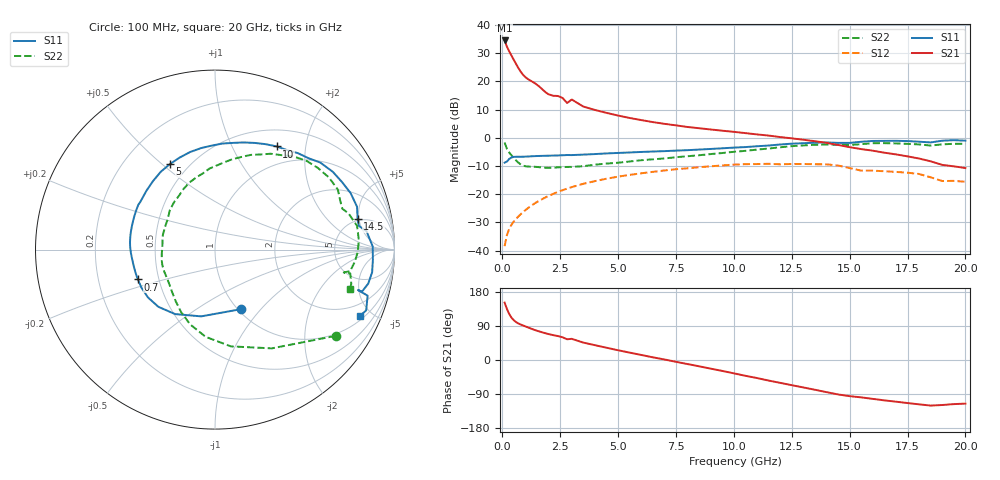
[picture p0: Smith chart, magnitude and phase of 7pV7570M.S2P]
! Infineon Technologies  Discrete & RF Semiconductors
! bfp620
! VCE = 0.75 V,  IC =  70 mA
! Common Emitter S-Parameters:  Sep 2002
# GHz  S  MA  R  50
!  f  S11  S21  S12  S22
! GHz  MAG  ANG  MAG  ANG  MAG  ANG  MAG  ANG
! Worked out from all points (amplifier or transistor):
!   59 points, 100 MHz to 20 GHz, reference 50 ohm
!   highest |S21| = 34.5 dB at 100 MHz (marker M1)
!   |S21| within 3 dB of that: start of sweep to 246.9 MHz
!   unconditionally stable (mu >= 1): 1.803 GHz to 2.397 GHz; 3.082 GHz to 10.85 GHz; 16.75 GHz to end of sweep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
!   at 1 GHz: K = 0.92, MSG = 23.6 dB, |S12| = -25.6 dB
!   at 5.5 GHz: K = 1.06, MAG = 8.6 dB, |S12| = -13.1 dB
!   at 20 GHz: K = 1.55, MAG = -1.9 dB, |S12| = -15.6 dB
!   S11 on the Smith chart (normalised r, x): 100 MHz: 1.03, -0.79; 700 MHz: 0.38, -0.16; 5 GHz: 0.40, +0.53; 10 GHz: 0.72, +1.51; 14.5 GHz: 4.73, +4.78; 20 GHz: 1.22, -4.30
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0.1  0.3623 -66.3  53.11 151.5  0.012 63.1  0.8257 -35.6
0.2  0.3799 -101.7  41.22 134.7  0.0189 58.7  0.6348 -60.1
0.3  0.4226 -121.8  33.89 121.3  0.0244 57.2  0.5463 -80.7
0.4  0.4484 -134.7  28.46 111.5  0.0289 56.7  0.4886 -96.2
0.5  0.4589 -144.5  23.95 104.6  0.033 56.7  0.439 -108.4
0.6  0.4614 -152.4  20.16 99.8  0.0368 57.0  0.3955 -118.6
0.7  0.4613 -158.9  17.09 96.3  0.0406 57.3  0.3608 -127.5
0.8  0.4611 -164.2  14.75 93.5  0.0444 57.6  0.3363 -135.3
1  0.4637 -172.1  11.85 88.6  0.0523 57.9  0.3131 -147.3
1.4  0.4734 177.6  9.312 79.3  0.0687 57.1  0.3062 -162.9
1.9  0.4804 165.5  6.278 70.0  0.0892 54.0  0.2944 178.7
2.8  0.495 149.7  4.137 54.7  0.1257 46.1  0.3042 157.2
3  0.4938 147.4  4.769 55.9  0.1337 44.2  0.3051 157.0
3.5  0.5036 139.3  3.579 45.9  0.1529 39.0  0.3138 146.9
5  0.5388 117.7  2.479 25.7  0.2051 23.0  0.3613 123.6
7  0.5801 91.6  1.769 1.4  0.2637 1.8  0.4301 99.0
10  0.6699 59.1  1.275 -35.2  0.3343 -32.0  0.5641 69.3
10.5  0.6846 54.0  1.211 -41.7  0.341 -38.6  0.5871 64.5
13.5  0.8186 22.6  0.87 -78.5  0.3403 -73.7  0.7514 32.3
14.5  0.8127 12.2  0.747 -90.9  0.3228 -88.9  0.7483 21.0
17  0.8845 -8.2  0.508 -110.0  0.2486 -104.4  0.7954 -1.0
20  0.8898 -24.4  0.291 -115.1  0.1661 -115.4  0.7821 -16.5
